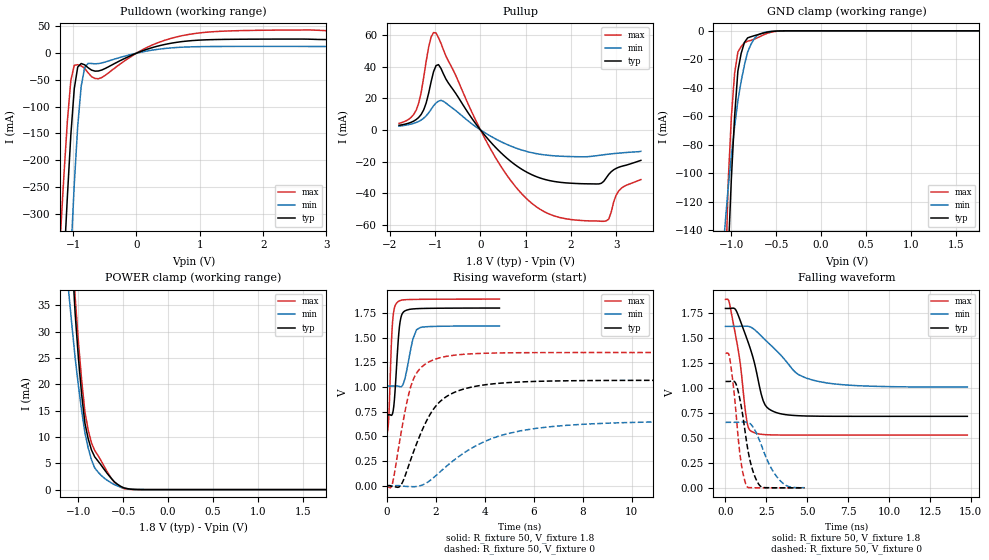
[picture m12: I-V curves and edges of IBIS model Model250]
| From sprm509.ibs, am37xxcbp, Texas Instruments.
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| Model based on original model for BQ18OMAPSMART1HYFBPB_SSBHV
|   Sub model PB_VS01L11_PUPD0_1P8
[model]   Model250
|[Input Load]   PI
|[Output Drive] SC01LB11
|Voltage   1.8V
|Mode   I/O
Model_type   I/O
Polarity   Non-Inverting
Enable   Active-Low
Vinl =  0.63
Vinh =  1.17
Cref =  15pF
Rref =  100.0000M
Vref =  0V
Vmeas =  0.9
C_comp   1.429432p   1.270657p   1.602015p
[Model Spec]
Vinl   0.63   0.567   0.6615
Vinh   1.17   1.053   1.2285
[Temperature Range]   25   125   -40
[Voltage Range]   1.8   1.62   1.89
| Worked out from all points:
|   slope of the pulldown table from 0 to 0.27 V, typ, clamps not added: 24.3 ohm
|   slope of the pullup table from 0 to 0.27 V, typ, clamps not added: 29.7 ohm
|   GND clamp passes 1 mA (typ) near -0.60 V on its own axis
|   POWER clamp passes 1 mA (typ) near -0.56 V on its own axis
|   rising waveform, R_fixture 50, V_fixture 1.8: 20-80 % time 176ps typ, 301ps min, 125ps max; typ from 0.717 V to 1.8 V
|   rising waveform, R_fixture 50, V_fixture 0: 20-80 % time 1.28ns typ, 2.76ns min, 683ps max; typ from 0 V to 1.07 V
|   falling waveform, R_fixture 50, V_fixture 1.8: 20-80 % time 1.08ns typ, 2.16ns min, 680ps max; typ from 1.8 V to 0.718 V
|   falling waveform, R_fixture 50, V_fixture 0: 20-80 % time 672ps typ, 1.09ns min, 499ps max; typ from 1.07 V to 0 V
[POWER_clamp]
-1.8V     362.5mA    191.4mA    412.8mA
-1.109V   56.69mA    37.71mA    60.38mA
-1.073V   44.6mA     31.22mA    47.8mA
-1.036V   33.44mA    25.04mA    36.59mA
-1V       24.98mA    19.72mA    28.06mA
-963.6mV  18.03mA    14.96mA    20.78mA
-927.3mV  12.59mA    10.77mA    14.74mA
-890.9mV  9.653mA    7.899mA    11.31mA
-818.2mV  6.214mA    4.114mA    7.414mA
-636.4mV  2.183mA    1.307mA    2.238mA
-418.2mV  83.85uA    105.2uA    35.14uA
1.764V    -1.228nA   -79.12nA   -1.453nA
[Pulldown]
-1.8V     -1.718A    -2.61A     -1.406A
-1.2V     -527.4mA   -844.5mA   -339.9mA
-1.145V   -396mA     -683.1mA   -229.1mA
-1.091V   -269mA     -526.7mA   -127.5mA
-1.036V   -153.6mA   -378.9mA   -51.17mA
-981.8mV  -66.34mA   -245.6mA   -22.67mA
-927.3mV  -26mA      -136.2mA   -21.54mA
-872.7mV  -19.34mA   -61.98mA   -23.69mA
-763.6mV  -27.2mA    -19.05mA   -36.72mA
-545.5mV  -31.39mA   -18.17mA   -45.46mA
872.7mV   23.46mA    11.88mA    35.92mA
3.545V    25.34mA    12.51mA    41.58mA
[Pullup]
-1.8V     2.903mA    2.423mA    4.112mA
-1.418V   6.595mA    4.711mA    12.64mA
-1.255V   12.69mA    7.42mA     33.23mA
-1.091V   30.4mA     13mA       58.69mA
-981.8mV  40.63mA    17.02mA    61.3mA
-818.2mV  35.38mA    18.12mA    50.59mA
272.7mV   -9.18mA    -4.728mA   -14.55mA
1.255V    -29.75mA   -15.09mA   -48.97mA
2.564V    -34.17mA   -16.31mA   -57.57mA
2.782V    -30.25mA   -15.5mA    -57.48mA
3.055V    -23.63mA   -14.68mA   -38.61mA
3.545V    -19.25mA   -13.56mA   -31.41mA
[GND_clamp]
-1.8V     -2.82A     -1.192A    -3.165A
-1.073V   -235.7mA   -138.4mA   -192.1mA
-1.036V   -159.5mA   -110.8mA   -107.5mA
-1V       -103.8mA   -87.85mA   -60.67mA
-963.6mV  -60mA      -67.28mA   -29.8mA
-927.3mV  -28.21mA   -49.08mA   -14.9mA
-890.9mV  -15.9mA    -35.48mA   -10.99mA
-854.5mV  -8.138mA   -24.07mA   -8.449mA
-818.2mV  -4.924mA   -14.85mA   -7.266mA
-709.1mV  -2.784mA   -3.064mA   -4.883mA
-563.6mV  -570.2uA   -404.5uA   -1.092mA
1.764V    -11.02pA   583.5nA    3.035nA
[Ramp]
dV/dt_f  0.6512825/1.085255n   0.3676745/2.175107n   0.8183042/0.6823778n
dV/dt_r  0.6507459/1.279391n   0.4007243/2.784082n   0.8225501/0.6841004n
R_load = 50
[Rising Waveform]
R_fixture = 50
V_fixture = 1.8
V_fixture_min = 1.62
V_fixture_max = 1.89
0s        717.2mV    1.009V     527.9mV
81ps      718.8mV    1.009V     718.7mV
225ps     727.1mV    1.009V     1.638V
306ps     871.3mV    1.009V     1.8V
405ps     1.252V     1.01V      1.852V
540ps     1.663V     1.002V     1.876V
747ps     1.772V     1.097V     1.884V
1.062ns   1.79V      1.485V     1.887V
1.359ns   1.795V     1.602V     1.888V
4.599ns   1.8V       1.618V     1.89V
[Rising Waveform]
R_fixture = 50
V_fixture = 0
V_fixture_min = 0
V_fixture_max = 0
0s        -233.5uV   109.6uV    -10.91mV
225ps     -8.714mV   -402.8uV   21.22mV
576ps     7.748mV    -1.677mV   530.4mV
846ps     173mV      -8.074mV   879.7mV
1.071ns   332mV      -10.33mV   1.072V
1.611ns   652.7mV    26.81mV    1.239V
2.106ns   836.6mV    125.2mV    1.292V
3.933ns   1.019V     440.7mV    1.341V
6.075ns   1.056V     580mV      1.348V
19.12ns   1.067V     655.8mV    1.349V
[Falling Waveform]
R_fixture = 50
V_fixture = 1.8
V_fixture_min = 1.62
V_fixture_max = 1.89
0s        1.8V       1.62V      1.89V
297ps     1.801V     1.62V      1.808V
837ps     1.707V     1.62V      1.323V
1.287ns   1.506V     1.622V     689.9mV
1.584ns   1.362V     1.609V     567.5mV
2.304ns   873.7mV    1.505V     535.5mV
3.231ns   749.1mV    1.357V     530.4mV
4.383ns   724.5mV    1.146V     529.8mV
5.787ns   718.8mV    1.064V     529.8mV
14.79ns   717.6mV    1.011V     529.8mV
[Falling Waveform]
R_fixture = 50
V_fixture = 0
V_fixture_min = 0
V_fixture_max = 0
0s        1.068V     657.3mV    1.349V
270ps     1.068V     657.7mV    1.289V
657ps     1.036V     657.5mV    727.8mV
927ps     849.8mV    659.5mV    283.5mV
1.287ns   463.9mV    660.1mV    20.35mV
1.656ns   178.8mV    616.9mV    1.545mV
2.16ns    13.37mV    442.3mV    170.5uV
2.745ns   1.369mV    213.2mV    17.36uV
3.339ns   336.9uV    72.78mV    2.735uV
4.833ns   45.61uV    1.646mV    380.6nV
